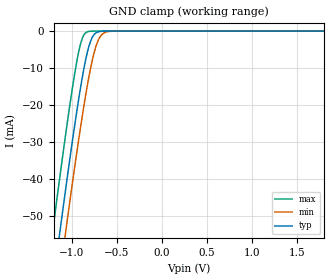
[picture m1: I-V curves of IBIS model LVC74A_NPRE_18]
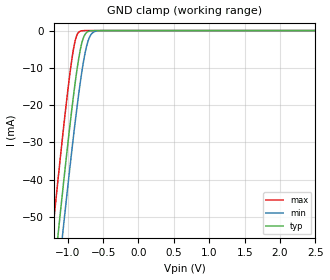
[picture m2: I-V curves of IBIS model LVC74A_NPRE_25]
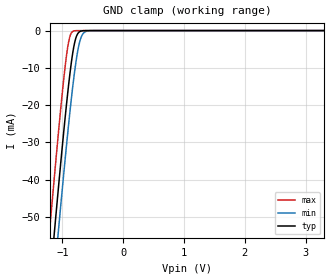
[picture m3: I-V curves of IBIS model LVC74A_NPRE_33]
| TEXAS INSTRUMENTS INCORPORATED
| Standard Linear and Logic Group
| IBIS Model of SN74LVC74A
| DUAL POSITIVE-EDGE-TRIGGERED D-TYPE FLIP-FLOPS WITH CLEAR AND PRESET
| This file contains package information for the following:
|  SOIC 14-pin (D) package as [Component] LVC74A_D
|  SSOP 14-pin (DB) package as [Component] LVC74A_DB
|  SOP 14-pin (NS) package as [Component] LVC74A_NS
|  TSSOP 14-pin (PW) package as [Component] LVC74A_PW
|   14-pin (RGY) package as [Componenet] LVC74A_RGY
| This device can be powered at the following Vccs:
|  1.8 volt Vcc
|  2.5 volt Vcc
|  3.3 volt Vcc
| This file provides unique models under the [Model Selector] for each Vcc.
| For operation at a specific Vcc, select the appropriate model after each
| [Model Selector] keyword.
[IBIS Ver]   3.2
[Comment char]  |_char
[File Name]   sn74lvc74a.ibs
[File Rev]   1.1 | b_die
[Date]   October 21, 2002
[Source]   Data created from TI-SPICE simulations at TI-SLL.
[Notes]   The following is an IBIS list for the LVC74A.
   Please contact sllibis@ti.com with questions and
   comments concerning SLL IBIS models.
   This IBIS model is created from a BA (back annotated netlist)
   -As there is no power clamp diode in the Input and Output
   Models, we removed the Pwr Clamp table data from those
   Models.
[Disclaimer] Property of Texas Instruments Incorporated.  Unauthorized
   reproduction and/or distribution is strictly prohibited.
   This product is protected under copyright law.
   Created  2002, (C) Copyright  2002, Texas Instruments
   Incorporated, All Rights Reserved
   UNLESS THERE IS A SIGNED, WRITTEN AGREEMENT TO THE
   CONTRARY, TEXAS INSTRUMENTS (TI) IS PROVIDING THE IBIS
   MODELS  AND WITHOUT ANY WARRANTY, EXPRESSED OR
   IMPLIED.  TI assumes no liability for:
   1) the accuracy of the IBIS models provided to your
   company;
   2) the proper functioning of these IBIS Models in your
   design or for any resulting applications; or
   3) infringement of patents, copyrights or intellectual
   property rights resulting from your use of these IBIS
   models.
   TI provides IBIS Models as a service to our customers.
   You and your company shall not distribute, sell or give
   these models to anyone else without prior written
   permission from TI.
   TI reserves the right to make changes to our products or
   to discontinue any semiconductor product or service
   without notice, and advises our customers to obtain the
   latest version of relevant information to verify, before
   placing orders, that the information being relied on is
   current.
   Please be aware that your receipt and use of the IBIS
   information provided shall serve as acceptance of these
   terms and conditions.  If you do not accept these terms,
   you should return or destroy the IBIS models and any
   other accompanying information immediately.
| Component LVC74A_D 14-pin SOIC
[Component]   LVC74A_D
[Manufacturer]   Texas Instruments, Inc.
[Package]
|   typ   min   max
R_pkg   3.100e-02   2.800e-02   3.400e-02
L_pkg   3.109e-09   2.462e-09   3.889e-09
C_pkg   4.730e-13   3.630e-13   6.280e-13
[Pin]   signal_name   model_name   R_pin   L_pin   C_pin
1   1NCLR   LVC74A_NCLR   3.300e-02   3.854e-09   6.220e-13
2   1D   LVC74A_IN   3.200e-02   3.188e-09   4.730e-13
3   1CLK   LVC74A_CLK   2.800e-02   2.462e-09   3.770e-13
4   1NPRE   LVC74A_NPRE   3.100e-02   2.596e-09   3.630e-13
5   1Q   LVC74A_OUT   2.800e-02   2.521e-09   3.720e-13
6   1NQ   LVC74A_OUT   3.400e-02   3.250e-09   4.760e-13
7   GND   GND   3.400e-02   3.889e-09   6.280e-13
8   2NQ   LVC74A_OUT   3.400e-02   3.889e-09   6.280e-13
9   2Q   LVC74A_OUT   3.400e-02   3.250e-09   4.760e-13
10   2NPRE   LVC74A_NPRE   2.800e-02   2.521e-09   3.720e-13
11   2CLK   LVC74A_CLK   3.100e-02   2.596e-09   3.640e-13
12   2D   LVC74A_IN   2.800e-02   2.462e-09   3.770e-13
13   2NCLR   LVC74A_NCLR   3.200e-02   3.188e-09   4.730e-13
14   VCC   POWER   3.300e-02   3.854e-09   6.220e-13
| Component LVC74A_DB 14-pin SSOP
[Component]   LVC74A_DB
[Manufacturer]   Texas Instruments, Inc.
[Package]
|   typ   min   max
R_pkg   4.400e-02   4.100e-02   4.600e-02
L_pkg   3.551e-09   3.258e-09   3.927e-09
C_pkg   4.020e-13   3.600e-13   4.210e-13
[Pin]   signal_name   model_name   R_pin   L_pin   C_pin
1   1NCLR   LVC74A_NCLR   4.600e-02   3.927e-09   4.080e-13
2   1D   LVC74A_IN   4.400e-02   3.587e-09   4.210e-13
3   1CLK   LVC74A_CLK   4.100e-02   3.289e-09   3.980e-13
4   1NPRE   LVC74A_NPRE   4.200e-02   3.258e-09   3.600e-13
5   1Q   LVC74A_OUT   4.100e-02   3.286e-09   4.030e-13
6   1NQ   LVC74A_OUT   4.400e-02   3.586e-09   4.210e-13
7   GND   GND   4.600e-02   3.927e-09   4.080e-13
8   2NQ   LVC74A_OUT   4.600e-02   3.927e-09   4.080e-13
9   2Q   LVC74A_OUT   4.400e-02   3.586e-09   4.210e-13
10   2NPRE   LVC74A_NPRE   4.100e-02   3.286e-09   4.030e-13
11   2CLK   LVC74A_CLK   4.300e-02   3.258e-09   3.600e-13
12   2D   LVC74A_IN   4.100e-02   3.289e-09   3.980e-13
13   2NCLR   LVC74A_NCLR   4.400e-02   3.587e-09   4.210e-13
14   VCC   POWER   4.600e-02   3.927e-09   4.080e-13
| Component LVC74A_NS 14-pin SOP
[Component]   LVC74A_NS
[Manufacturer]   Texas Instruments, Inc.
[Package]
|   typ   min   max
R_pkg   4.500e-02   3.900e-02   5.400e-02
L_pkg   3.796e-09   2.561e-09   4.952e-09
C_pkg   5.280e-13   2.880e-13   7.100e-13
[Pin]   signal_name   model_name   R_pin   L_pin   C_pin
1   1NCLR   LVC74A_NCLR   4.700e-02   4.867e-09   7.060e-13
2   1D   LVC74A_IN   5.100e-02   4.083e-09   5.920e-13
3   1CLK   LVC74A_CLK   4.100e-02   2.915e-09   3.760e-13
4   1NPRE   LVC74A_NPRE   3.900e-02   2.561e-09   2.880e-13
5   1Q   LVC74A_OUT   4.100e-02   3.101e-09   4.300e-13
6   1NQ   LVC74A_OUT   4.700e-02   4.047e-09   5.890e-13
7   GND   GND   5.100e-02   4.909e-09   7.000e-13
8   2NQ   LVC74A_OUT   4.500e-02   4.784e-09   6.940e-13
9   2Q   LVC74A_OUT   5.400e-02   4.176e-09   5.970e-13
10   2NPRE   LVC74A_NPRE   3.900e-02   3.287e-09   4.490e-13
11   2CLK   LVC74A_CLK   3.900e-02   2.586e-09   2.940e-13
12   2D   LVC74A_IN   4.000e-02   2.802e-09   3.710e-13
13   2NCLR   LVC74A_NCLR   4.900e-02   4.080e-09   5.930e-13
14   VCC   POWER   5.200e-02   4.952e-09   7.100e-13
| Component LVC74A_PW 14-pin TSSOP
[Component]   LVC74A_PW
[Manufacturer]   Texas Instruments, Inc.
[Package]
|   typ   min   max
R_pkg   3.200e-02   2.900e-02   3.500e-02
L_pkg   2.378e-09   2.170e-09   2.680e-09
C_pkg   3.140e-13   2.700e-13   3.350e-13
[Pin]   signal_name   model_name   R_pin   L_pin   C_pin
1   1NCLR   LVC74A_NCLR   3.300e-02   2.618e-09   3.300e-13
2   1D   LVC74A_IN   3.100e-02   2.313e-09   3.170e-13
3   1CLK   LVC74A_CLK   3.000e-02   2.310e-09   3.140e-13
4   1NPRE   LVC74A_NPRE   3.100e-02   2.173e-09   2.720e-13
5   1Q   LVC74A_OUT   3.000e-02   2.204e-09   3.090e-13
6   1NQ   LVC74A_OUT   3.200e-02   2.315e-09   3.170e-13
7   GND   GND   3.500e-02   2.680e-09   3.350e-13
8   2NQ   LVC74A_OUT   3.300e-02   2.640e-09   3.330e-13
9   2Q   LVC74A_OUT   3.400e-02   2.347e-09   3.190e-13
10   2NPRE   LVC74A_NPRE   2.900e-02   2.277e-09   3.130e-13
11   2CLK   LVC74A_CLK   3.100e-02   2.170e-09   2.700e-13
12   2D   LVC74A_IN   3.100e-02   2.244e-09   3.110e-13
13   2NCLR   LVC74A_NCLR   3.300e-02   2.343e-09   3.210e-13
14   VCC   POWER   3.500e-02   2.657e-09   3.320e-13
| Component LVC74A_RGY 14-pin
[Component]   LVC74A_RGY
[Manufacturer]   Texas Instruments, Inc.
[Package]
|   typ   min   max
R_pkg   0.029   0.023   0.041
L_pkg   0.773e-09   0.657e-09   0.998e-09
C_pkg   0.136e-12   0.115e-12   0.156e-12
[Pin]   signal_name   model_name   R_pin   L_pin   C_pin
1   1NCLR   LVC74A_NCLR   0.027   0.831e-09   0.130e-12
2   1D   LVC74A_IN   0.027   0.866e-09   0.135e-12
3   1CLK   LVC74A_CLK   0.041   0.998e-09   0.156e-12
4   1NPRE   LVC74A_NPRE   0.031   0.767e-09   0.142e-12
5   1Q   LVC74A_OUT   0.031   0.765e-09   0.142e-12
6   1NQ   LVC74A_OUT   0.031   0.783e-09   0.144e-12
7   GND   GND   0.031   0.781e-09   0.137e-12
8   2NQ   LVC74A_OUT   0.023   0.657e-09   0.115e-12
9   2Q   LVC74A_OUT   0.023   0.814e-09   0.129e-12
10   2NPRE   LVC74A_NPRE   0.028   0.704e-09   0.129e-12
11   2CLK   LVC74A_CLK   0.027   0.672e-09   0.136e-12
12   2D   LVC74A_IN   0.027   0.696e-09   0.138e-12
13   2NCLR   LVC74A_NCLR   0.027   0.725e-09   0.140e-12
14   VCC   POWER   0.030   0.763e-09   0.136e-12
| Model LVC74A_NPRE
[Model Selector]   LVC74A_NPRE
LVC74A_NPRE_18   1.8 volt Vcc
LVC74A_NPRE_25   2.5 volt Vcc
LVC74A_NPRE_33   3.3 volt Vcc
| Model LVC74A_CLK
[Model Selector]   LVC74A_CLK
LVC74A_CLK_18   1.8 volt Vcc
LVC74A_CLK_25   2.5 volt Vcc
LVC74A_CLK_33   3.3 volt Vcc
| Model LVC74A_NCLR
[Model Selector]   LVC74A_NCLR
LVC74A_NCLR_18   1.8 volt Vcc
LVC74A_NCLR_25   2.5 volt Vcc
LVC74A_NCLR_33   3.3 volt Vcc
| Model LVC74A_IN
[Model Selector]   LVC74A_IN
LVC74A_IN_18   1.8 volt Vcc
LVC74A_IN_25   2.5 volt Vcc
LVC74A_IN_33   3.3 volt Vcc
| Model LVC74A_OUT
[Model Selector]   LVC74A_OUT
LVC74A_OUT_18   1.8 volt Vcc
LVC74A_OUT_25   2.5 volt Vcc
LVC74A_OUT_33   3.3 volt Vcc
| Models and submodels in the file (15): LVC74A_NPRE_18 (Input), LVC74A_NPRE_25 (Input), LVC74A_NPRE_33 (Input), LVC74A_CLK_18 (Input), LVC74A_CLK_25 (Input), LVC74A_CLK_33 (Input), LVC74A_NCLR_18 (Input), LVC74A_NCLR_25 (Input), LVC74A_NCLR_33 (Input), LVC74A_IN_18 (Input), LVC74A_IN_25 (Input), LVC74A_IN_33 (Input), LVC74A_OUT_18 (Output), LVC74A_OUT_25 (Output), LVC74A_OUT_33 (Output)
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[Model]   LVC74A_NPRE_18
Model_type  Input
Vinl=0.5775
Vinh=1.2675
| variable   typ   min   max
C_comp   4.98pF   4.16pF   5.98pF
[Temperature Range]   40   100   -40
| Ambient temperature   25   85   -40
[Voltage range]   1.8   1.65   1.95
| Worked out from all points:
|   GND clamp passes 1 mA (typ) near -0.75 V on its own axis
[GND Clamp]
| LVC74A_NPRE_18
|   Voltage   I(typ)   I(min)   I(max)
-5.5V     -915.9mA   -925.7mA   -903.9mA
-1.215V   -69.33mA   -80.91mA   -54.47mA
-1.135V   -54.61mA   -66.2mA    -39.73mA
-1.075V   -43.82mA   -55.36mA   -29.01mA
-1.055V   -40.28mA   -51.8mA    -25.54mA
-955mV    -23.31mA   -34.48mA   -9.608mA
-885mV    -12.72mA   -23.13mA   -2.077mA
-825mV    -5.482mA   -14.34mA   -191.7uA
-780mV    -2.057mA   -8.704mA   -23.97uA
-715mV    -287.1uA   -2.975mA   -1.13uA
-650mV    -30.77uA   -620.5uA   -53.02nA
1.8V      3.327pA    7.106pA    3.026pA
[Model]   LVC74A_NPRE_25
Model_type  Input
Vinl=0.7
Vinh=1.7
| variable   typ   min   max
C_comp   4.85pF   3.85pF   5.98pF
[Temperature Range]   40   100   -40
| Ambient temperature   25   85   -40
[Voltage range]   2.5   2.3   2.7
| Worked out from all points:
|   GND clamp passes 1 mA (typ) near -0.75 V on its own axis
[GND Clamp]
| LVC74A_NPRE_25
|   Voltage   I(typ)   I(min)   I(max)
-5.5V     -915.9mA   -925.7mA   -903.9mA
-1.215V   -69.33mA   -80.91mA   -54.47mA
-1.14V    -55.53mA   -67.11mA   -40.64mA
-1.075V   -43.82mA   -55.36mA   -29.01mA
-1.06V    -41.16mA   -52.69mA   -26.4mA
-960mV    -24.12mA   -35.32mA   -10.31mA
-885mV    -12.72mA   -23.13mA   -2.077mA
-830mV    -5.985mA   -15.02mA   -239.8uA
-780mV    -2.057mA   -8.704mA   -23.97uA
-720mV    -339uA     -3.291mA   -1.43uA
-650mV    -30.77uA   -620.5uA   -53.02nA
2.5V      4.714pA    8.54pA     4.389pA
[Model]   LVC74A_NPRE_33
Model_type  Input
Vinl=0.8
Vinh=2.0
| variable   typ   min   max
C_comp   4.73pF   3.67pF   6.06pF
[Temperature Range]   40   100   -40
| Ambient temperature   25   85   -40
[Voltage range]   3.3   3   3.6
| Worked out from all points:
|   GND clamp passes 1 mA (typ) near -0.75 V on its own axis
[GND Clamp]
| LVC74A_NPRE_33
|   Voltage   I(typ)   I(min)   I(max)
-5.5V     -915.9mA   -925.7mA   -903.9mA
-1.225V   -71.19mA   -82.77mA   -56.33mA
-1.145V   -56.44mA   -68.03mA   -41.55mA
-1.12V    -51.89mA   -63.47mA   -37.02mA
-1.08V    -44.71mA   -56.26mA   -29.89mA
-1.06V    -41.16mA   -52.69mA   -26.4mA
-965mV    -24.94mA   -36.16mA   -11.03mA
-885mV    -12.72mA   -23.13mA   -2.077mA
-780mV    -2.057mA   -8.704mA   -23.97uA
-715mV    -287.1uA   -2.975mA   -1.13uA
-640mV    -21.7uA    -472.6uA   -33.12nA
3.3V      11.73pA    10.22pA    5.93pA
